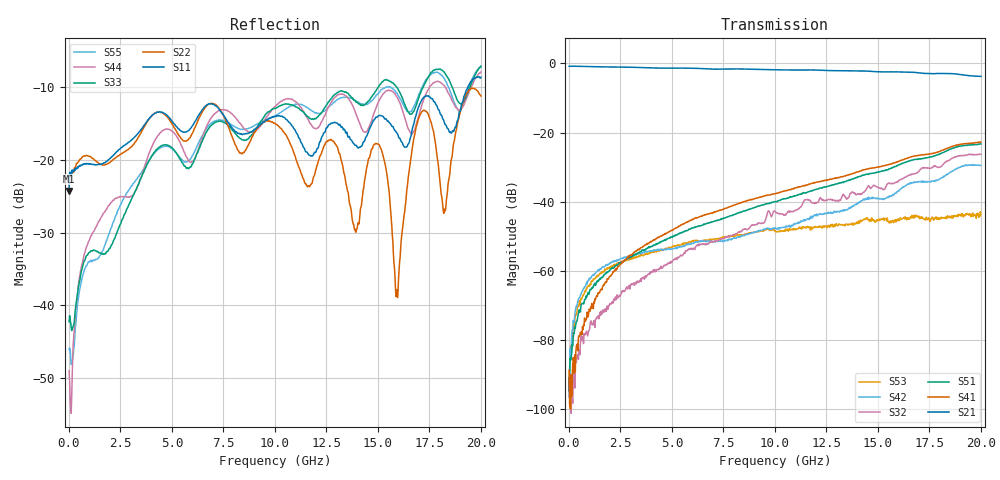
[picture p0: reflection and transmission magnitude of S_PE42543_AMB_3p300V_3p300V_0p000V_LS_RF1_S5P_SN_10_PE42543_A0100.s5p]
!Agilent Technologies,N5230C,MY49001593,A.09.33.09
!Agilent N5230C: A.09.33.09
!Date: Friday, March 21, 2014 07:22:33
!Correction: S11(Full 5 Port(1,2,3,5,6))
!S12(Full 5 Port(1,2,3,5,6))
!S13(Full 5 Port(1,2,3,5,6))
!S15(Full 5 Port(1,2,3,5,6))
!S16(Full 5 Port(1,2,3,5,6))
!S21(Full 5 Port(1,2,3,5,6))
!S22(Full 5 Port(1,2,3,5,6))
!S23(Full 5 Port(1,2,3,5,6))
!S25(Full 5 Port(1,2,3,5,6))
!S26(Full 5 Port(1,2,3,5,6))
!S31(Full 5 Port(1,2,3,5,6))
!S32(Full 5 Port(1,2,3,5,6))
!S33(Full 5 Port(1,2,3,5,6))
!S35(Full 5 Port(1,2,3,5,6))
!S36(Full 5 Port(1,2,3,5,6))
!S51(Full 5 Port(1,2,3,5,6))
!S52(Full 5 Port(1,2,3,5,6))
!S53(Full 5 Port(1,2,3,5,6))
!S55(Full 5 Port(1,2,3,5,6))
!S56(Full 5 Port(1,2,3,5,6))
!S61(Full 5 Port(1,2,3,5,6))
!S62(Full 5 Port(1,2,3,5,6))
!S63(Full 5 Port(1,2,3,5,6))
!S65(Full 5 Port(1,2,3,5,6))
!S66(Full 5 Port(1,2,3,5,6))
!S5P File: Measurements: <S11,S12,S13,S15,S16>,
!<S21,S22,S23,S25,S26>,
!<S31,S32,S33,S35,S36>,
!<S51,S52,S53,S55,S56>,
!<S61,S62,S63,S65,S66>:
# Hz S  dB  R 50
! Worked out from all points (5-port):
!   801 points, 10 MHz to 20 GHz, reference 50 ohm
!   strongest paths, dB at 10 MHz, 5.008 GHz, 10.01 GHz, 15 GHz, 20 GHz:
!     S21: -0.8, -1.3, -1.8, -2.4, -3.7
!     S41: -88.8, -48.2, -37.7, -30.0, -22.7
!     S51: -94.7, -50.2, -39.9, -31.4, -23.2
!     S32: -91.7, -57.4, -42.7, -35.8, -26.3
!     S42: -96.5, -53.6, -47.6, -39.0, -29.5
!     S53: -94.7, -53.0, -48.6, -45.2, -43.6
!   lowest |S11| = -24.2 dB at 10 MHz (marker M1), VSWR 1.13, Z = 56.3 - j1.84 ohm
!   |S11| at or under -10 dB: start of sweep to 19.36 GHz
